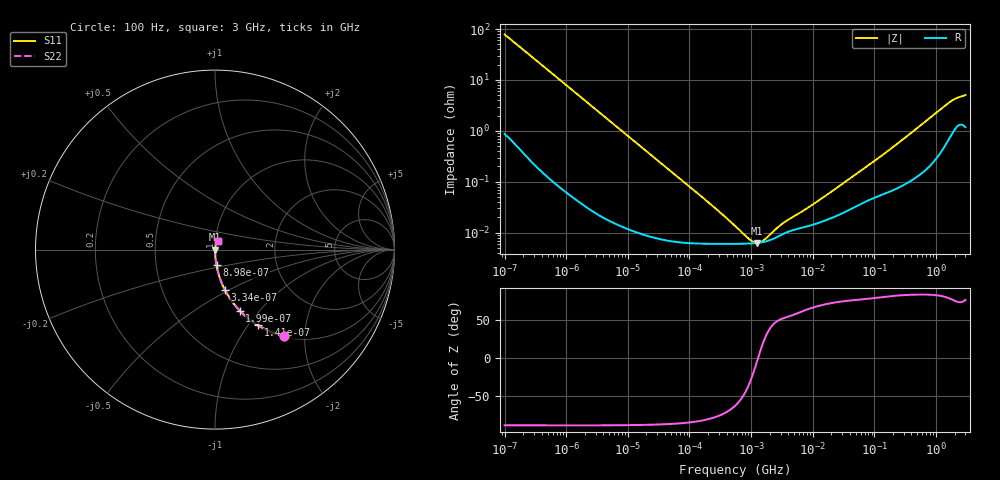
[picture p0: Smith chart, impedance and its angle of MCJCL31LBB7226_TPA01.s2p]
! MCJCL31LBB7226_TPA01  S-PARAMETER MODEL  ( Standard Model )
! Model Generated by TAIYO YUDEN Corporation (http://www.ty-top.com)
! Version 2.0
! TAIYO YUDEN Control No. 240604
! Copyright(c) 2015 TAIYO YUDEN CO.,LTD. All Rights Reserved.
! Product Description (link to TY-COMPAS)
! https://ds.yuden.co.jp/TYCOMPAS/or/detail?pn=MCJCL31LBB7226KTPA01&u=M
! Products Name : Multilayer Ceramic Capacitors
! Characteristics :
!  Capacitance : 22 [uF] , Rated Voltage : 10 [V] , TCC : X7R
!  Case Size : 3.2 x 1.6 / 0.126 x 0.063 [mm/inch] , Thickness : 1.6 / 0.063 [mm/inch]
!  (Conditions: Temperature = 25 [degC] , DC Bias Voltage = 0 [V])
! External Node Assignments :
!  1  o---| |---o  2
! GND o---------o GND
! Frequency Range : 100Hz  -  3GHz  [ 401 STEP ]
# MHZ S RI R 50
! Freq[MHz].  S11 Real  S11 Imag  S21 Real  S21 Imag  S12 Real  S12 Imag  S22 Real  S22 Imag
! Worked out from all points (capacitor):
!   401 points, 100 Hz to 3 GHz, reference 50 ohm
!   read as one part in series: C = 20.3 uF near 109 Hz
!   lowest |Z| = 6.32 mohm at 1.241 MHz (marker M1)
!   series resonance near 1.299 MHz, so ESL is about 740 pH
!   S11 on the Smith chart (normalised r, x): 100 Hz: 1.02, -1.57; 141 Hz: 1.01, -1.11; 199 Hz: 1.01, -0.79; 334 Hz: 1.00, -0.47; 898 Hz: 1.00, -0.18; 3 GHz: 1.02, +0.10
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0.0001  0.3818 -0.4803  0.6182 0.4803  0.6182 0.4803  0.3818 -0.4803
0.000141  0.2392 -0.4214  0.7608 0.4214  0.7608 0.4214  0.2392 -0.4214
0.000199  0.1377 -0.34  0.8623 0.34  0.8623 0.34  0.1377 -0.34
0.000334  0.0547 -0.2233  0.9453 0.2233  0.9453 0.2233  0.0547 -0.2233
0.000559  0.0207 -0.1384  0.9793 0.1384  0.9793 0.1384  0.0207 -0.1384
0.000898  0.0084 -0.0875  0.9916 0.0875  0.9916 0.0875  0.0084 -0.0875
0.001788  0.00234 -0.0444  0.9977 0.0444  0.9977 0.0444  0.00234 -0.0444
0.005476  0.000375 -0.0146  0.9996 0.0146  0.9996 0.0146  0.000375 -0.0146
0.031977  8.19e-05 -0.00252  0.9999 0.00252  0.9999 0.00252  8.19e-05 -0.00252
0.21248  6.06e-05 -0.000371  0.9999 0.000371  0.9999 0.000371  6.06e-05 -0.000371
0.547723  6.04e-05 -0.000122  0.9999 0.000122  0.9999 0.000122  6.04e-05 -0.000122
0.650627  6.05e-05 -9.37e-05  0.9999 9.37e-05  0.9999 9.37e-05  6.05e-05 -9.37e-05
0.740304  6.07e-05 -7.43e-05  0.9999 7.43e-05  0.9999 7.43e-05  6.07e-05 -7.43e-05
1.240863  6.29e-05 -5.76e-06  0.9999 5.76e-06  0.9999 5.76e-06  6.29e-05 -5.76e-06
2.171352  7.38e-05 6.68e-05  0.9999 -6.68e-05  0.9999 -6.68e-05  7.38e-05 6.68e-05
3.486191  9.74e-05 0.000129  0.9999 -0.000129  0.9999 -0.000129  9.74e-05 0.000129
9.794414  0.000142 0.000322  0.9999 -0.000322  0.9999 -0.000322  0.000142 0.000322
74.05258  0.000417 0.00192  0.9996 -0.00192  0.9996 -0.00192  0.000417 0.00192
175.1444  0.000653 0.00419  0.9993 -0.00419  0.9993 -0.00419  0.000653 0.00419
1642.185  0.00827 0.035  0.9917 -0.035  0.9917 -0.035  0.00827 0.035
2126.076  0.0132 0.0412  0.9868 -0.0412  0.9868 -0.0412  0.0132 0.0412
3000  0.014 0.0482  0.986 -0.0482  0.986 -0.0482  0.014 0.0482
